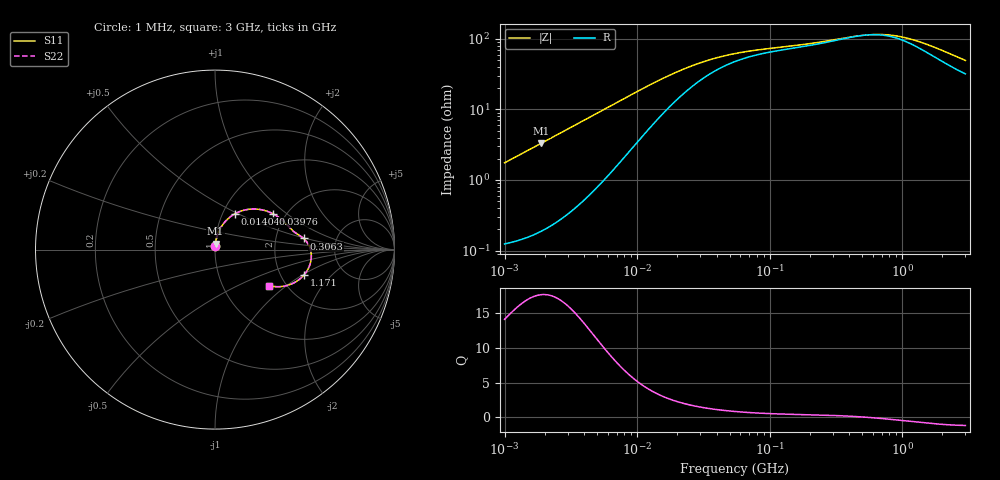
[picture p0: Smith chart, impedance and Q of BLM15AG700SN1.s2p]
! BLM15AG700SN1
# Hz S RI R 50
!Freq.(Hz) S11(Real) S11(Imag) S21(Real) S21(Imag) S12(Real) S12(Imag) S22(Real) S22(Imag)
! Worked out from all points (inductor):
!   401 points, 1 MHz to 3 GHz, reference 50 ohm
!   read as one part in series: L = 279 nH near 1.041 MHz
!   highest Q = 17.6 at 1.897 MHz (marker M1), where L = 279 nH
!   self-resonance near 534.5 MHz
!   S11 on the Smith chart (normalised r, x): 1 MHz: 1.00, +0.03; 14.04 MHz: 1.14, +0.48; 39.76 MHz: 1.72, +0.80; 306.3 MHz: 2.89, +0.48; 1.171 GHz: 2.70, -1.03; 3 GHz: 1.64, -0.76
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1000000  0.00154 0.0174  0.9985 -0.0174  0.9985 -0.0174  0.00154 0.0174
1897447  0.00298 0.0331  0.997 -0.0331  0.997 -0.0331  0.00298 0.0331
3823119  0.00927 0.0664  0.9907 -0.0664  0.9907 -0.0664  0.00927 0.0664
8017732  0.0392 0.1337  0.9608 -0.1337  0.9608 -0.1337  0.0392 0.1337
1.061086e7  0.0674 0.1674  0.9326 -0.1674  0.9326 -0.1674  0.0674 0.1674
1.404268e7  0.1102 0.1992  0.8898 -0.1992  0.8898 -0.1992  0.1102 0.1992
1.461624e7  0.1176 0.2031  0.8824 -0.2031  0.8824 -0.2031  0.1176 0.2031
1.858443e7  0.1666 0.2208  0.8334 -0.2208  0.8334 -0.2208  0.1666 0.2208
2.362996e7  0.2203 0.2263  0.7797 -0.2263  0.7797 -0.2263  0.2203 0.2263
3.065274e7  0.2765 0.218  0.7235 -0.218  0.7235 -0.218  0.2765 0.218
3.976269e7  0.3245 0.1988  0.6755 -0.1988  0.6755 -0.1988  0.3245 0.1988
5.477226e7  0.3689 0.1689  0.6311 -0.1689  0.6311 -0.1689  0.3689 0.1689
1.018679e8  0.4197 0.1182  0.5803 -0.1182  0.5803 -0.1182  0.4197 0.1182
2.094008e8  0.4637 0.0835  0.5363 -0.0835  0.5363 -0.0835  0.4637 0.0835
3.062963e8  0.4933 0.0622  0.5067 -0.0622  0.5067 -0.0622  0.4933 0.0622
5.473095e8  0.5329 -0.00364  0.4671 0.00364  0.4671 0.00364  0.5329 -0.00364
8.005644e8  0.5328 -0.0698  0.4672 0.0698  0.4672 0.0698  0.5328 -0.0698
1.171007e9  0.4975 -0.1394  0.5025 0.1394  0.5025 0.1394  0.4975 -0.1394
1.519029e9  0.4525 -0.178  0.5475 0.178  0.5475 0.178  0.4525 -0.178
1.893158e9  0.4049 -0.1991  0.5951 0.1991  0.5951 0.1991  0.4049 -0.1991
2.359433e9  0.3536 -0.2069  0.6464 0.2069  0.6464 0.2069  0.3536 -0.2069
3e9  0.3001 -0.2008  0.6999 0.2008  0.6999 0.2008  0.3001 -0.2008
